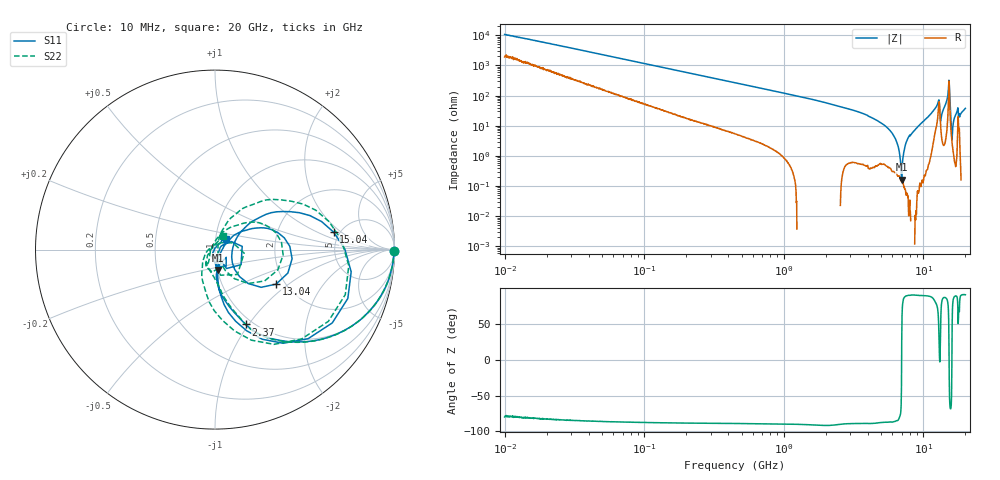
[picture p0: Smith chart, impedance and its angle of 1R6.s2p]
!Keysight Technologies,P5008B,MY61100088,A.16.20.02
!Date: Monday, October 30, 2023 16:21:19
!Correction: S11(C  2-Port  )
!S21(C  2-Port  )
!S12(C  2-Port  )
!S22(C  2-Port  )
!S2P File: Measurements: S11, S21, S12, S22:Log Frequency Sweep
# Hz S  dB  R 50
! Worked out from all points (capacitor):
!   1601 points, 10 MHz to 20 GHz, reference 50 ohm
!   read as one part in series: C = 1.48 pF near 10.39 MHz
!   lowest |Z| = 161 mohm at 7 GHz (marker M1)
!   series resonance near 6.986 GHz, so ESL is about 350 pH
!   S11 on the Smith chart (normalised r, x): 10 MHz: open; 2.37 GHz: 0.93, -0.97; 13.04 GHz: 1.80, -0.82; 15.04 GHz: 4.47, +1.56; 20 GHz: 1.12, +0.14
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1e7  -0.01 -0.5  -40.60 79.2  -40.61 79.1  -0.01 -0.5
3.555162e7  -0.03 -1.8  -30.16 83.3  -30.16 83.3  -0.03 -1.8
1.263918e8  -0.09 -6.3  -19.47 81.5  -19.48 81.5  -0.09 -6.3
4.472136e8  -0.62 -20.9  -9.20 67.9  -9.21 67.9  -0.62 -21.0
1.589917e9  -4.20 -54.9  -2.00 35.7  -2.00 35.8  -4.20 -55.2
2.369619e9  -6.92 -67.7  -0.94 23.0  -0.94 23.0  -7.02 -68.0
5.652411e9  -15.70 -86.7  -0.13 -0.7  -0.14 -0.7  -15.76 -90.5
6.999632e9  -18.79 -82.4  -0.05 -6.5  -0.06 -6.5  -18.90 -107.6
9.003717e9  -21.82 -87.6  -0.00 -14.4  -0.01 -14.4  -22.20 -117.2
1.053187e10  -28.91 -24.2  0.01 -20.9  0.00 -20.9  -33.26 172.8
1.249622e10  -11.09 25.8  -1.20 -35.0  -1.20 -35.0  -11.90 37.1
1.273595e10  -8.77 14.8  -2.26 -37.5  -2.27 -37.5  -9.64 21.9
1.304209e10  -8.15 -29.4  -3.68 -15.4  -3.69 -15.4  -9.71 -32.3
1.374174e10  -17.12 28.7  -0.24 -27.7  -0.25 -27.7  -18.10 68.5
1.447892e10  -9.23 34.6  -0.77 -41.5  -0.77 -41.5  -9.36 48.8
1.503978e10  -3.49 8.3  -4.58 -61.9  -4.59 -62.0  -3.68 13.7
1.577149e10  -8.90 -77.9  -1.18 -4.7  -1.18 -4.7  -9.35 -90.7
1.62275e10  -16.04 -84.4  -0.28 -18.0  -0.28 -18.1  -16.73 -120.2
1.685609e10  -25.27 -71.4  -0.11 -26.7  -0.11 -26.8  -25.90 -162.8
1.810106e10  -19.10 -55.9  -0.86 -28.8  -0.87 -28.8  -17.95 -96.7
1.90721e10  -45.18 127.4  -0.05 -36.6  -0.05 -36.6  -35.69 149.1
2e10  -21.26 44.0  -0.03 -41.9  -0.03 -41.9  -21.26 59.4
